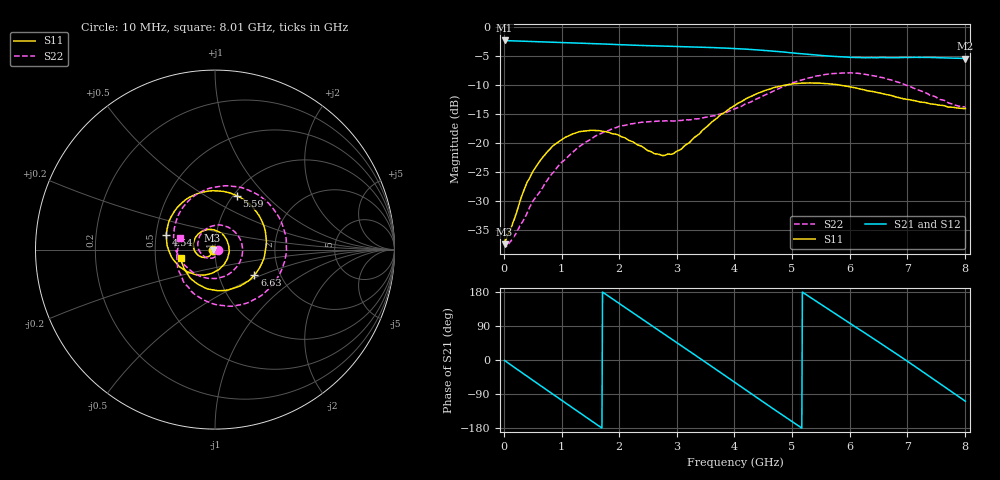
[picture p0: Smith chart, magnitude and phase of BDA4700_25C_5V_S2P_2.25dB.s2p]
!Agilent Technologies,E5071B,MY42404982,A.09.10
!Date: Mon Oct 20 13:27:01 2025
!Data & Calibration Information:
!Freq	S11:SOLT2(ON)	S21:SOLT2(ON)	S12:SOLT2(ON)	S22:SOLT2(ON)
# Hz S RI R 50
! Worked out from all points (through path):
!   801 points, 10 MHz to 8.01 GHz, reference 50 ohm
!   highest |S21| = -2.36 dB at 10 MHz (marker M1); lowest = -5.5 dB at 8.01 GHz (marker M2)
!   group delay of S21, straight-line fit = 286 ps
!   lowest |S11| = -37.4 dB at 10 MHz (marker M3), VSWR 1.03, Z = 48.7 - j0.175 ohm
!   |S11| at or under -10 dB: start of sweep to 4.909 GHz; 5.799 GHz to end of sweep
!   |S22| runs from -37.8 to -7.9 dB; largest |S21 - S12| = 0.0056
!   S11 on the Smith chart (normalised r, x): 10 MHz: 0.97, -0.00; 4.54 GHz: 0.57, +0.10; 5.59 GHz: 1.04, +0.70; 6.63 GHz: 1.48, -0.45; 8.01 GHz: 0.68, -0.07
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1e7  -0.0133 -0.00179  0.7618 -0.0162  0.7617 -0.0173  0.0141 -0.00155
3.3e8  -0.0239 -0.0289  0.6107 -0.4355  0.6108 -0.4363  0.0164 -0.0137
7.2e8  -0.0679 -0.0431  0.1692 -0.7204  0.1692 -0.7205  -0.00731 -0.0448
1.02e9  -0.1066 -0.0181  -0.2306 -0.6945  -0.2311 -0.6947  -0.0553 -0.0417
1.35e9  -0.1199 0.0378  -0.577 -0.4343  -0.5772 -0.4342  -0.0949 0.0167
1.64e9  -0.0935 0.0873  -0.7084 -0.082  -0.7089 -0.0821  -0.0764 0.0897
1.92e9  -0.0425 0.1116  -0.6503 0.2705  -0.6507 0.2704  -0.00516 0.1343
2.32e9  0.0356 0.0892  -0.3038 0.6219  -0.3032 0.622  0.1153 0.0942
2.68e9  0.0756 0.0257  0.132 0.671  0.1319 0.6707  0.1525 -0.0226
3.36e9  0.0131 -0.1154  0.661 0.0983  0.662 0.0979  -0.0081 -0.1609
3.67e9  -0.0734 -0.1416  0.6039 -0.2666  0.6041 -0.268  -0.104 -0.1372
4.01e9  -0.1819 -0.1069  0.331 -0.5594  0.3317 -0.5591  -0.185 -0.0665
4.54e9  -0.2712 0.083  -0.2627 -0.5663  -0.2623 -0.5669  -0.224 0.131
4.95e9  -0.188 0.2565  -0.5527 -0.2311  -0.5531 -0.2327  -0.1161 0.2985
5.35e9  -0.000904 0.3278  -0.5466 0.1777  -0.5472 0.1764  0.1082 0.3514
5.59e9  0.123 0.3002  -0.417 0.3758  -0.4172 0.3762  0.2493 0.2984
6.09e9  0.2802 0.1048  0.0158 0.5429  0.0169 0.5446  0.3977 0.0165
6.63e9  0.2198 -0.1413  0.4465 0.3074  0.4473 0.3067  0.2357 -0.2689
6.68e9  0.2043 -0.159  0.4716 0.2668  0.4727 0.266  0.2078 -0.2843
7.25e9  -0.0194 -0.2234  0.4768 -0.2645  0.4764 -0.2654  -0.0947 -0.2612
7.64e9  -0.1405 -0.1554  0.1851 -0.5056  0.1847 -0.5067  -0.2071 -0.1068
8.01e9  -0.1919 -0.0491  -0.1716 -0.5036  -0.1711 -0.5041  -0.194 0.0634
